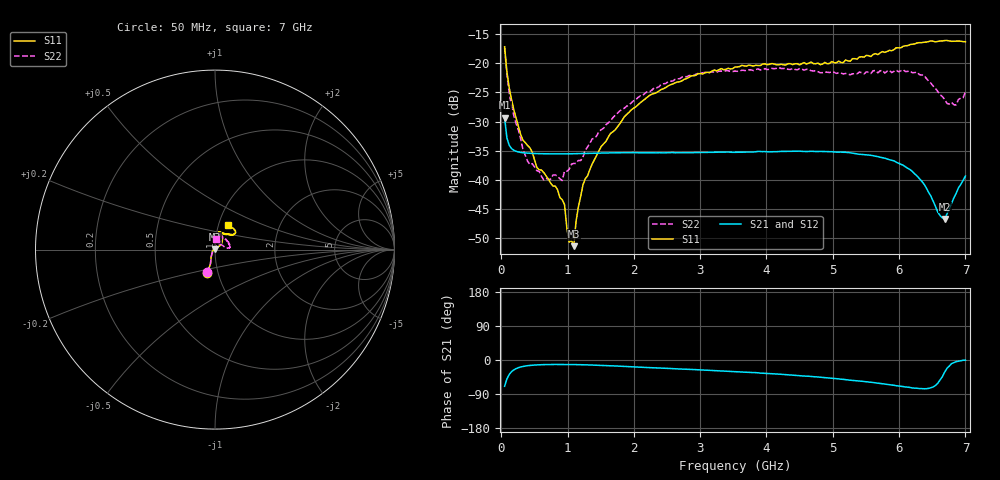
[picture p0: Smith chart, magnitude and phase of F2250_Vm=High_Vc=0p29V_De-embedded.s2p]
! Integrated Device Technology
! Corporate Headquarters
! 6024 Silver Creek Valley Road
! San Jose, CA 95138  USA
! Phone:  1-408-284-8200
! Toll Free:  1-800-223-1366
! Webpage:  http://www.idt.com/
! Timing and RF Division
! 515 Groton Road, Suite 102
! Westford, MA 01886-6024
! Device:  F2250
! Description: Voltage Variable RF Attenuator
! Frequency:  50.0 -  6000.00 MHz
! Package:  3x3 mm Thin QFN Plastic Package: 16 pin
! Ports:  2 RF, 3 DC
!  Pin  1  = GND
!  Pin  2  = NC
!  Pin  3  = RF1  = Port 1
!  Pin  4  = NC
!  Pin  5  = GND
!  Pin  6  = GND
!  Pin  7  = GND
!  Pin  8  = GND
!  Pin  9  = NC
!  Pin 10  = RF2  = Port 2
!  Pin 11  = NC
!  Pin 12  = GND
!  Pin 13  = GND
!  Pin 14  = VCNTRL
!  Pin 15  = VDD
!  Pin 16  = VMODE
! Vcntrl:  0.290 Volts
! Vmode:  +3.300 Volts
! Vdd:  +3.30  Volts
! Current:  1.251 mA
! Data:  The device was measured on a the F2250 evaluation board which has
!  individual transmission lines to the RF pins.  Data was collected
!  using a calibrated network analyzer.  The evaluation board was
!  de-embedded using a TRL calibration technique.
!  The reference plane is the edge of the package pin.
! Misc:  SN 10
!  Action Tracker AT0258
! Date Measured:  2014-11-26
! Date:  2015-10-15  MJV
! Note:
!  Integrated Device Technology supplies this data as a sample of measured
!  data at the package pin for this product.  Your particular data for this
!  product may vary.
!  Data was taken at 25 degrees C.
!  Integrated Device Technology reserves the right to change this data at anytime.
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# GHz S dB R 50
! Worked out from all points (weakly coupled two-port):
!   201 points, 50 MHz to 7 GHz, reference 50 ohm
!   highest |S21| = -29.37 dB at 50 MHz (marker M1); lowest = -46.7 dB at 6.687 GHz (marker M2)
!   lowest |S11| = -51.4 dB at 1.093 GHz (marker M3), VSWR 1.01, Z = 50 + j0.27 ohm
!   |S11| at or under -10 dB: start of sweep to end of sweep
!   |S22| runs from -40.1 to -17.4 dB; largest |S21 - S12| = 5.8e-05
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0.05  -17.18 -108.5  -29.37 -69.3  -29.36 -69.3  -17.44 -110.3
0.08475  -21.47 -107.4  -32.83 -49.9  -32.83 -49.9  -21.96 -108.3
0.189  -28.00 -120.0  -34.93 -26.1  -34.93 -26.1  -29.01 -122.7
0.29325  -32.27 -127.4  -35.30 -18.4  -35.30 -18.4  -33.03 -130.8
0.3975  -34.12 -142.1  -35.43 -15.0  -35.43 -15.0  -36.83 -155.9
0.5365  -37.89 -154.5  -35.50 -12.9  -35.50 -12.9  -38.44 -179.3
0.64075  -38.75 -162.5  -35.53 -12.2  -35.53 -12.2  -40.01 158.8
0.91875  -43.40 156.0  -35.55 -11.8  -35.55 -11.8  -40.13 123.0
0.9535  -44.24 171.3  -35.55 -11.8  -35.55 -11.8  -38.53 119.7
1.023  -50.69 139.8  -35.54 -11.9  -35.54 -11.9  -38.22 102.6
1.0925  -51.38 89.6  -35.53 -12.1  -35.52 -12.0  -37.19 93.5
1.12725  -47.17 61.9  -35.51 -12.2  -35.51 -12.2  -37.19 86.2
1.2315  -40.87 40.9  -35.48 -12.5  -35.48 -12.5  -36.12 72.1
1.6485  -32.02 41.2  -35.39 -15.2  -35.39 -15.3  -29.90 57.5
2.37825  -24.76 46.6  -35.35 -21.1  -35.36 -21.1  -24.04 52.6
3.525  -20.65 71.7  -35.27 -30.8  -35.28 -30.8  -21.36 72.3
4.7065  -20.06 72.0  -35.12 -44.1  -35.12 -44.1  -21.33 70.0
5.85325  -17.79 40.5  -36.54 -65.0  -36.54 -65.1  -21.22 22.8
6.27025  -16.53 39.4  -39.33 -74.5  -39.33 -74.7  -21.54 8.0
6.68725  -16.11 47.9  -46.71 -32.0  -46.69 -31.7  -26.20 27.9
6.861  -16.22 54.5  -42.30 -4.4  -42.26 -4.4  -27.15 57.5
7  -16.32 62.4  -39.36 -0.7  -39.32 -0.8  -24.94 84.1
